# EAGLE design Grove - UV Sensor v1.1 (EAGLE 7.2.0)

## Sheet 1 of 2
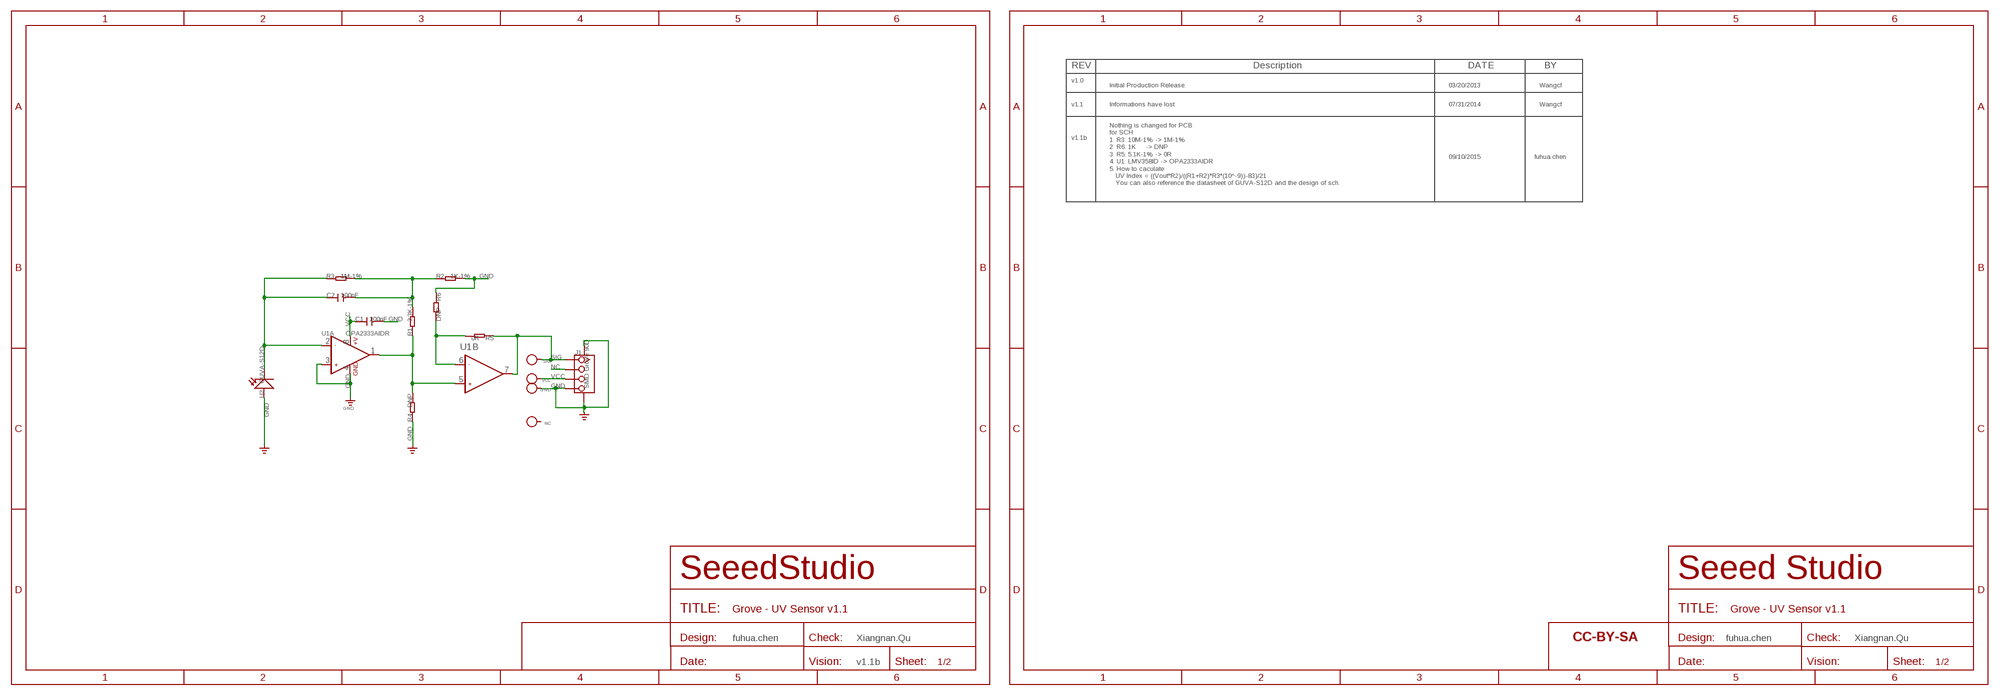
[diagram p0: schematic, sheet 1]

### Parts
C1  100nF  C-0603  [C0603]
C2  100nF  C-0603  [C0603]
GND  PAD-TEST-POINT'4545'  [TP_4545]
J1  SMD Grove 90D  TWIG-4P-2.0-SMD-FEMALE-REINFORCE'DD'  [4P-SMD-2.0]
NC  PAD-TEST-POINT'4545'  [TP_4545]
R1  3.3K-1%  R-0603  [R0603]
R2  1K-1%  R-0603  [R0603]
R3  1M-1%  R-0603  [R0603]
R4  DNP  R-0603  [R0603]
R5  0R  R-0603  [R0603]
R6  DNP  R-0603  [R0603]
SIG  PAD-TEST-POINT'4545'  [TP_4545]
U1  OPA2333AIDR  LMV358D  [SO08]
U2  GUVA-S12D  PHOTODIODE  [LED-3528]
U$30  SEEEDSTUDIO-OPEN-SCH-FRAME  [SEEEDSTUDIO-PCB-FRAME]
VCC  PAD-TEST-POINT'4545'  [TP_4545]

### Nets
GND: C1.2 GND.T J1.4 J1.SS1 J1.SS2 R2.2 R4.1 R6.1 U1.3(A:+IN1) U1.4(A:GND) U2.1(+)
N$1: C2.1 R3.1 U1.2(A:-IN1) U2.2(-)
N$2: R5.2 R6.2 U1.6(B:-IN2)
N$3: C2.2 R1.2 R2.1 R3.2
N$4: J1.1 R5.1 SIG.T U1.7(B:OUT2)
NC: J1.2
SIG: R1.1 R4.2 U1.1(A:OUT1) U1.5(B:+IN2)
VCC: C1.1 J1.3 U1.8(A:+V) VCC.T
Unconnected: NC.T

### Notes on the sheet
- REV | Description | DATE | BY
- v1.0
- Initial Production Release. | 03/20/2013 | Wangcf
- v1.1 | Informations have lost | 07/31/2014 | Wangcf
- v1.1b
- 09/10/2015 | fuhua.chen
- Nothing is changed for PCB
  for SCH:
  1. R3: 10M-1% -> 1M-1%
  2. R6: 1K     -> DNP
  3. R5: 5.1K-1% -> 0R
  4. U1: LMV358ID -> OPA2333AIDR
  5. How to caculate:
     UV Index = ((Vout*R2)/((R1+R2)*R3*(10^-9))-83)/21
     You can also reference the datasheet of GUVA-S12D and the design of sch.
- fuhua.chen | Xiangnan.Qu | fuhua.chen | Xiangnan.Qu
- v1.1b

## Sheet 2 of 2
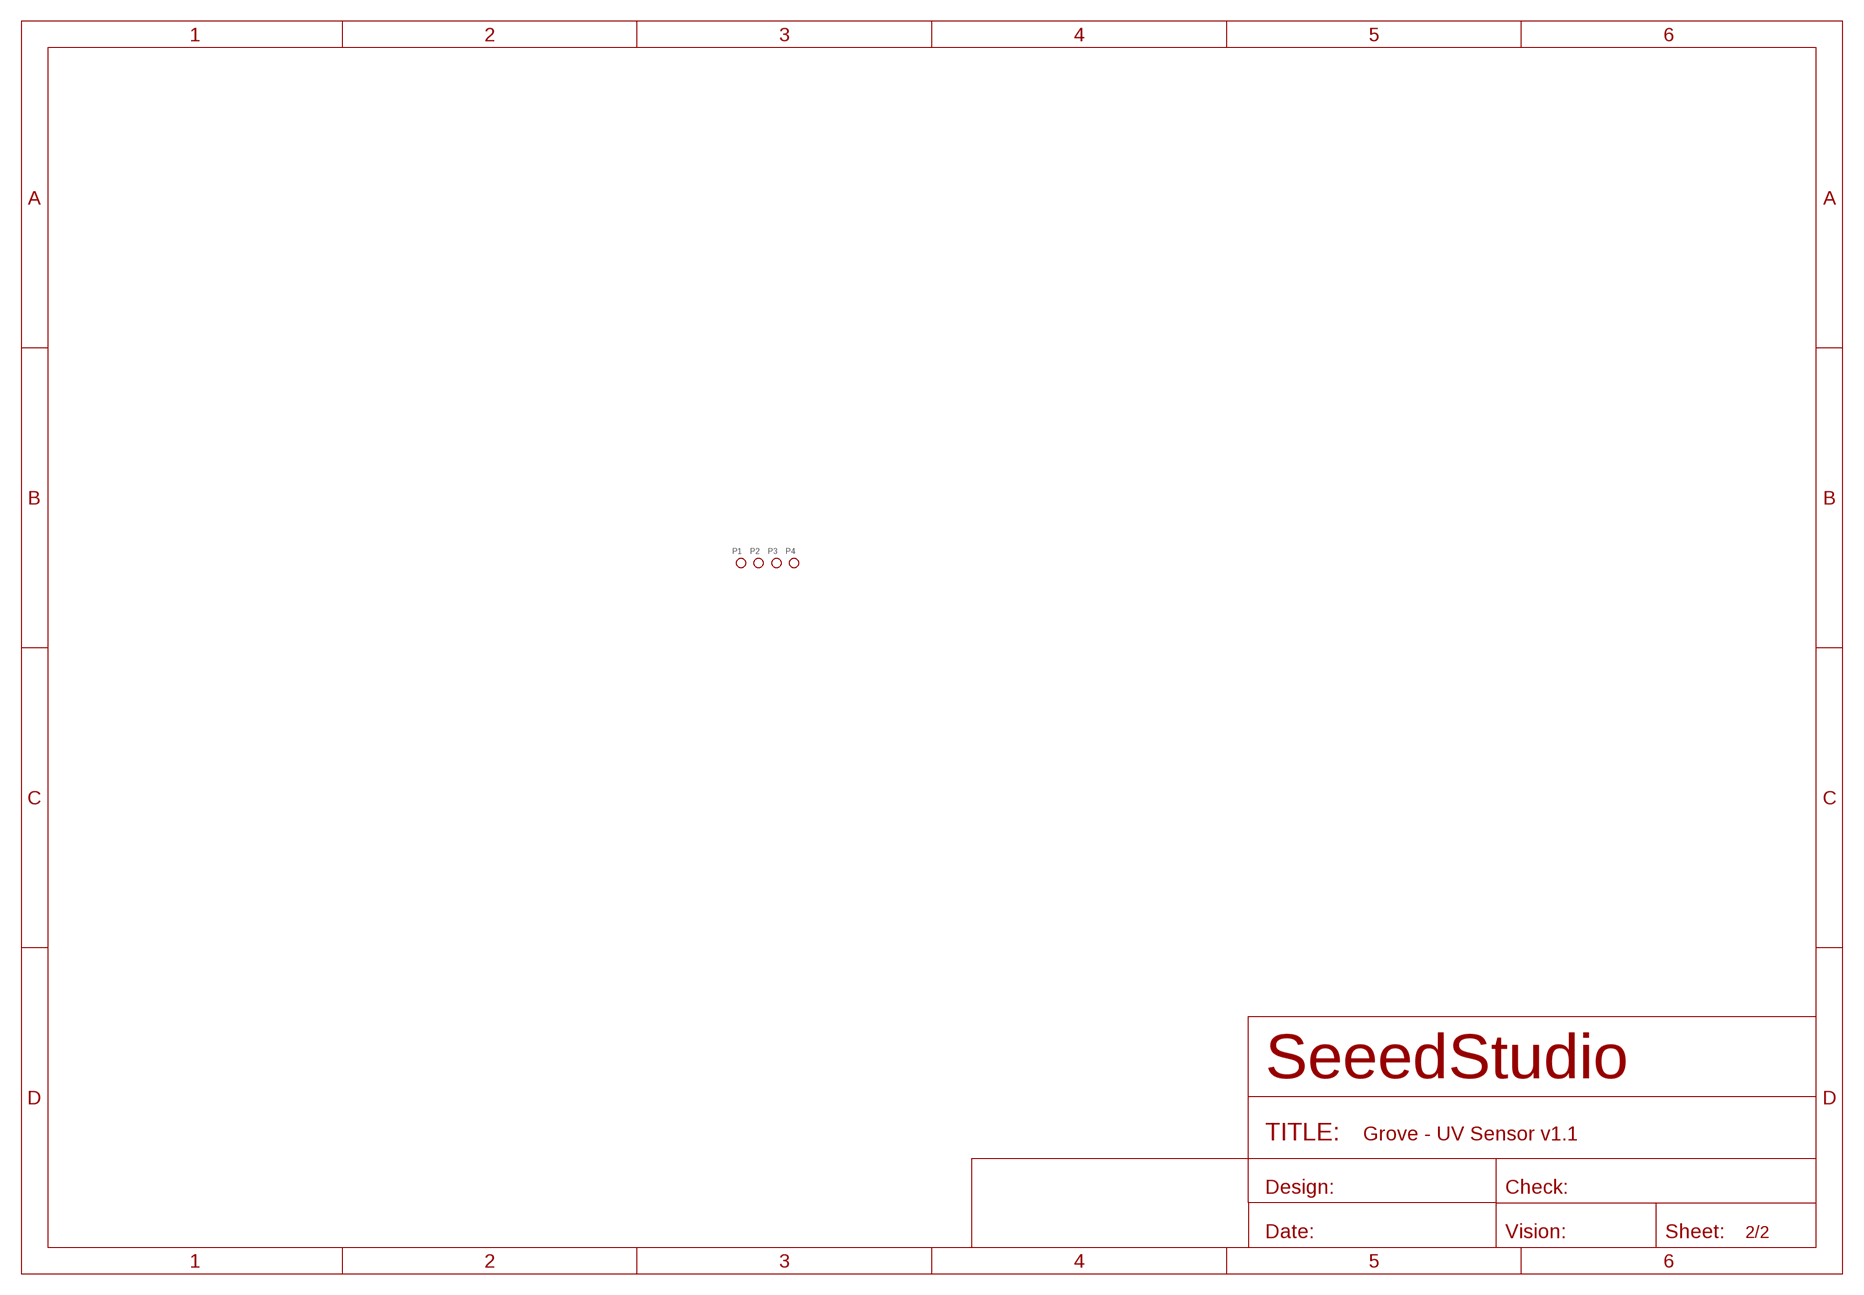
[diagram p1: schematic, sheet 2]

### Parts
P1  PAD-MARK  [ROUND-MARK-1.0]
P2  PAD-MARK  [ROUND-MARK-1.0]
P3  PAD-MARK  [ROUND-MARK-1.0]
P4  PAD-MARK  [ROUND-MARK-1.0]

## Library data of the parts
C1 C2 = Discrete:C*: Ceramic Capacitors
GND NC SIG VCC = Discrete:PAD-TEST-POINT; PARTNO: DNP
J1 = Connector:TWIG-4P-2.0-SMD-FEMALE-REINFORCE
P1-P4 = Discrete:PAD-MARK; PARTNO: DNP
R1-R6 = Discrete:R*
U1 = IC:LMV358: General purpose LOW Voltage, Rail-to-Rail Output Amplifiers http://www.fairchildsemi.com/ds/LM/LMV358.pdf
U2 = Test:PHOTODIODE
U$30 = moudle-new:SEEEDSTUDIO-OPEN-SCH-FRAME

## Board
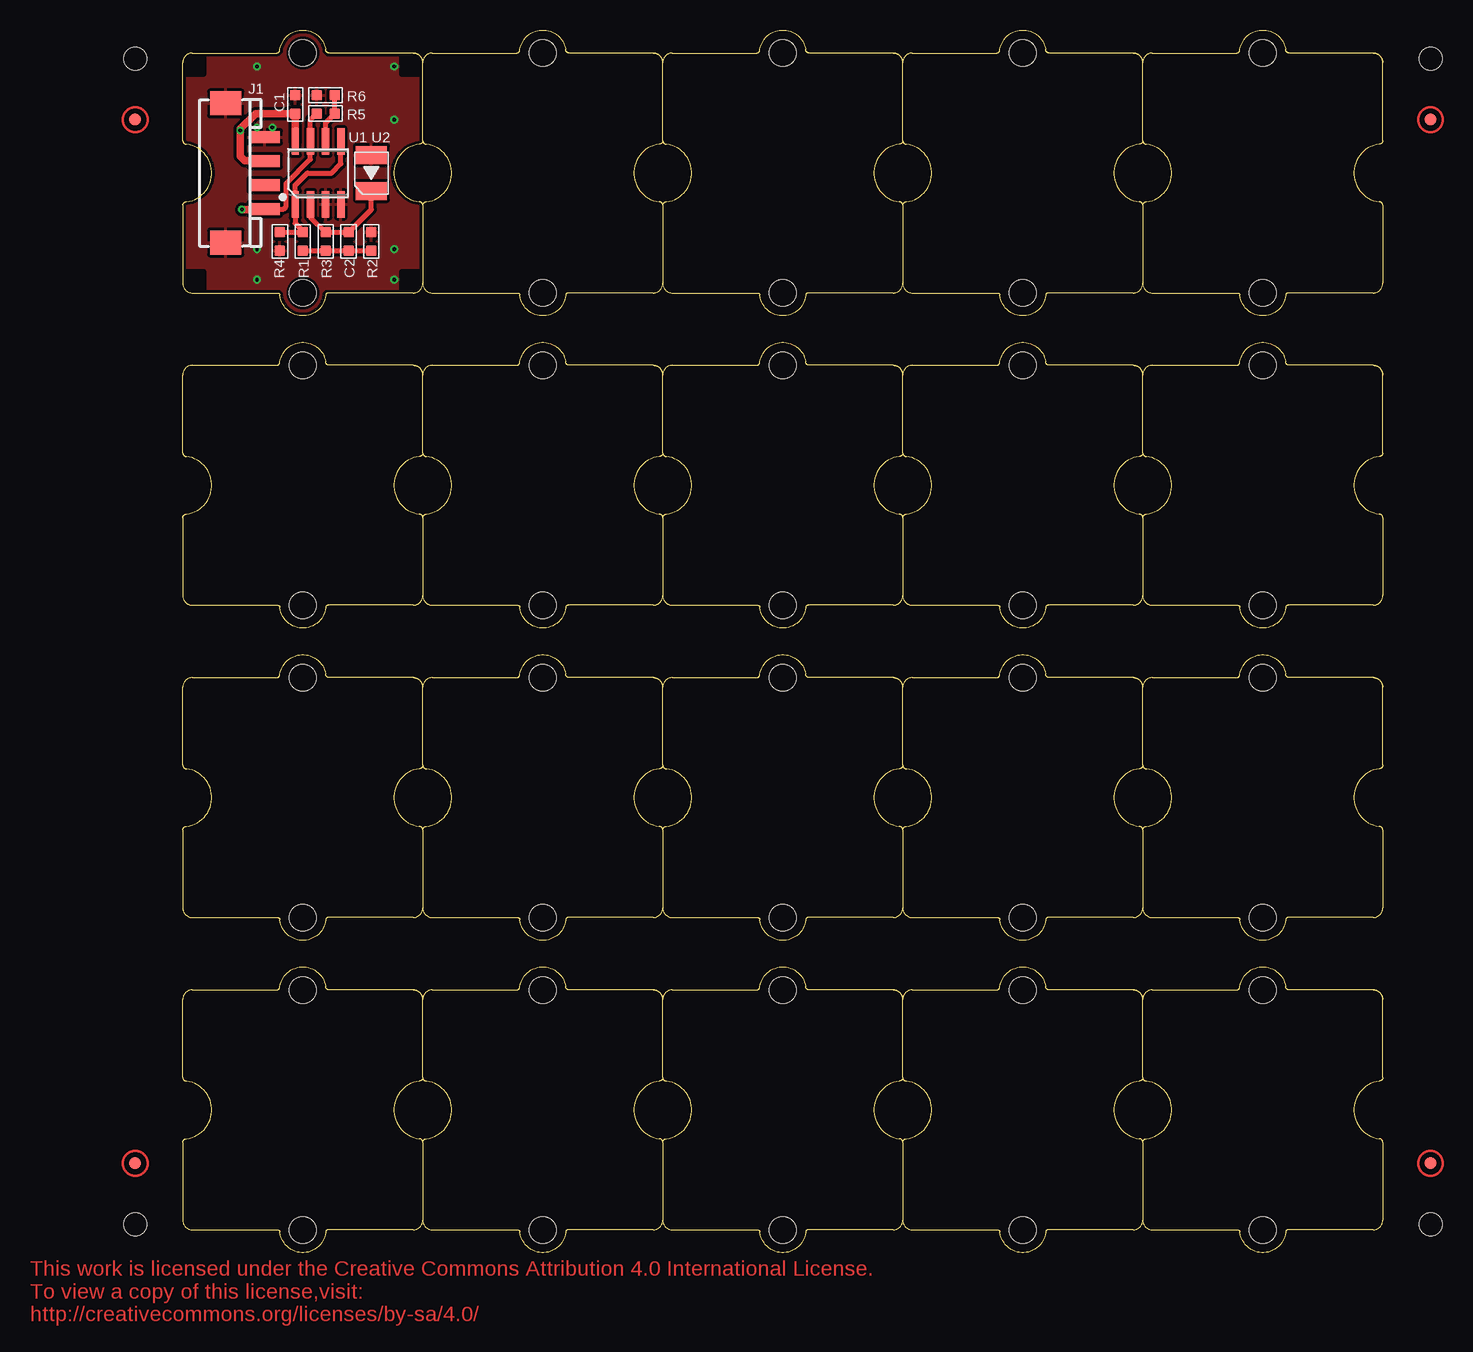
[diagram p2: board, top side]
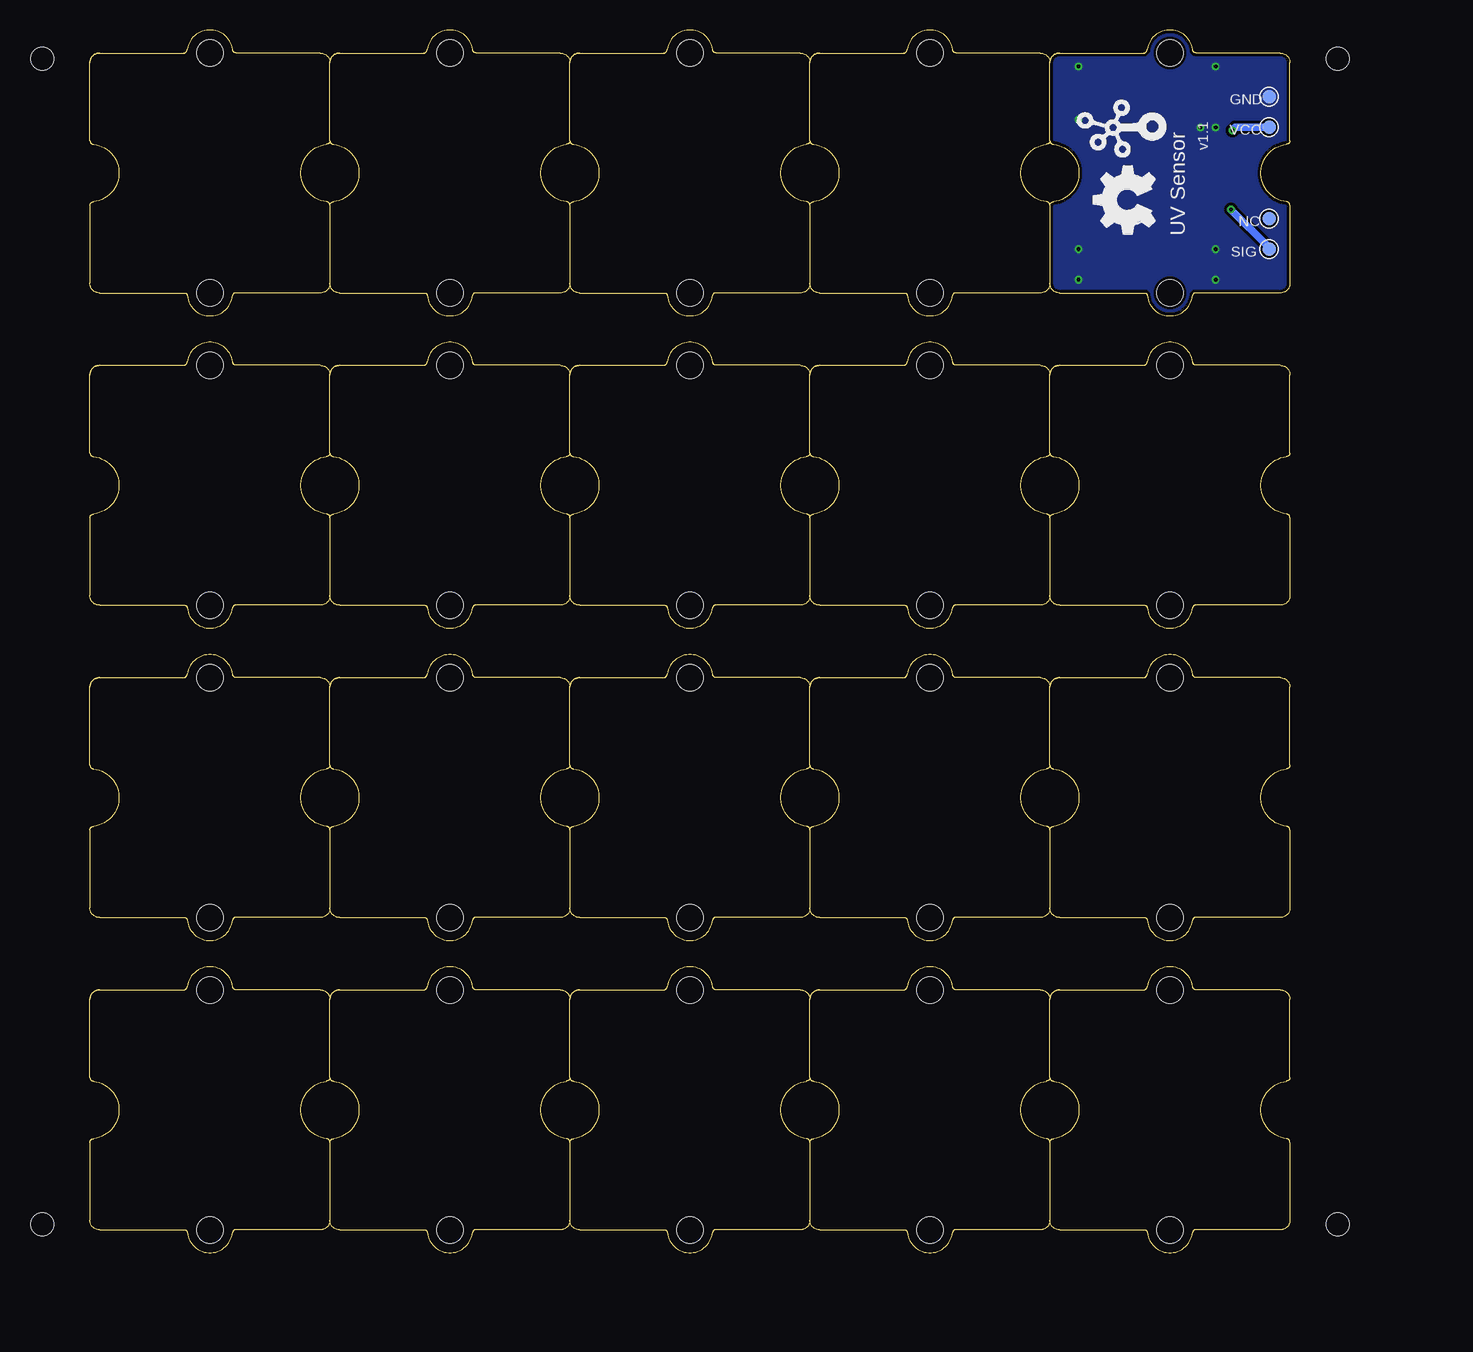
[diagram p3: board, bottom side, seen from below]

Size 100 x 101.93 mm. Coordinates in mm from the lower left corner, seen from the top.
Copper layers (1*16): Top 0.035mm / dielectric 1.5mm / Bottom 0.035mm
Design rules "SeeedStudio_rule_no_angle_090911 *": minimum track width 6mil, minimum drill 12mil, track to track 6mil, track to pad 6mil, pad to pad 6mil, via to via 6mil, smd to smd 0mil, copper to edge 10mil, drill to drill 10mil, minimum pad ring 10mil, minimum via ring 6mil, stop-mask expansion 2mil, vias tented up to drill 25mil, thermal gap 10mil
Holes 1.91 mm at -3.97,2.38 -3.97,99.54 103.98,99.54 103.98,2.38

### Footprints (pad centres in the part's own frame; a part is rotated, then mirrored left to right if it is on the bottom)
C0603 = smd 0.889 x 0.889: 1 -0.762,0; 2 0.762,0
TP_4545 = smd 1.143 x 1.143: T 0,0
4P-SMD-2.0 = smd 1 x 2.54: 1 -3,0; 2 -1,0; 3 1,0; 4 3,0 | smd 2 x 2.6: SS1 -5.8,3.25; SS2 5.8,3.25
ROUND-MARK-1.0 = smd 1.016 x 1.016: P$1 0,0
R0603 = smd 0.889 x 0.889: 1 -0.762,0; 2 0.762,0
SO08 = smd 0.61 x 2.21: 1 -1.905,-2.616; 2 -0.635,-2.616; 3 0.635,-2.616; 4 1.905,-2.616; 5 1.905,2.616; 6 0.635,2.616; 7 -0.635,2.616; 8 -1.905,2.616
LED-3528 = smd 1.5 x 2.6: 1 -1.5,0; 2 1.5,0
1U-DIM-W/-DRILL = hole 2.2: 0,-10; 0,10

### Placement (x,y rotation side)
C1  9.37,95.73 90 top
C2  13.81,84.3 270 top
GND  1.74,96.36 270 bottom
J1  6.83,90.01 90 top
NC  1.74,86.2 270 bottom
P1  not placed on the board
P2  not placed on the board
P3  not placed on the board
P4  not placed on the board
R1  10,84.3 270 top
R2  15.71,84.3 90 top
R3  11.9,84.3 270 top
R4  8.1,84.3 90 top
R5  11.9,94.97 0 top
R6  11.9,96.49 0 top
SIG  1.74,83.66 270 bottom
U1  11.27,90.01 0 top
U2  15.71,90.01 270 top
U$1  [1U-DIM-W/-DRILL]  10,90.01 0 top
U$3  [OSHW_FILLX200_NOTEXT]  11.27,84.93 90 bottom
U$4  [TWIGLOGO]  11.27,93.82 90 bottom
U$10  [1U-DIM-W/-DRILL]  10,90.01 0 top
U$11  [1U-DIM-W/-DRILL]  30,90.01 0 top
U$12  [1U-DIM-W/-DRILL]  50,90.01 0 top
U$13  [1U-DIM-W/-DRILL]  70,90.01 0 top
U$14  [1U-DIM-W/-DRILL]  90,90.01 0 top
U$15  [1U-DIM-W/-DRILL]  30,63.98 0 top
U$16  [1U-DIM-W/-DRILL]  50,63.98 0 top
U$17  [1U-DIM-W/-DRILL]  70,63.98 0 top
U$18  [1U-DIM-W/-DRILL]  90,63.98 0 top
U$19  [1U-DIM-W/-DRILL]  10,63.98 0 top
U$20  [1U-DIM-W/-DRILL]  30,37.94 0 top
U$21  [1U-DIM-W/-DRILL]  50,37.94 0 top
U$22  [1U-DIM-W/-DRILL]  70,37.94 0 top
U$23  [1U-DIM-W/-DRILL]  90,37.94 0 top
U$24  [1U-DIM-W/-DRILL]  10,37.94 0 top
U$25  [1U-DIM-W/-DRILL]  30,11.91 0 top
U$26  [1U-DIM-W/-DRILL]  50,11.91 0 top
U$27  [1U-DIM-W/-DRILL]  70,11.91 0 top
U$28  [1U-DIM-W/-DRILL]  90,11.91 0 top
U$29  [1U-DIM-W/-DRILL]  10,11.91 0 top
U$30  not placed on the board
VCC  1.74,93.82 270 bottom

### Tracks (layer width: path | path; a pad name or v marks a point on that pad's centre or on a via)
GND  (via drill 0.3 pad 0.64)
  other vias: 6.19,93.82 6.19,81.12 6.19,98.9 6.19,83.66 17.62,98.9 17.62,94.46 17.62,81.12 17.62,83.66 7.46,93.82
  pour Top (isolate 0.254): -2.19,102.08 21.43,102.08 21.43,76.68 -2.19,76.68
  pour Bottom (isolate 0.254): -2.19,102.08 -2.19,76.68 21.43,76.68 21.43,102.08
N$1
  Top 0.406: U1.2 10.63,86.33 R3.1 C2.1 15.71,86.97 U2.2
N$2
  Top 0.406: U1.6 11.9,94.2 R5.2 R6.2
N$3
  Top 0.406: R3.2 R1.2 C2.2 R2.1
N$4  (via drill 0.3)
  Top 0.406: R5.1 10.63,94.46 U1.7 10.63,91.16 8.6,89.12 8.6,87.22 8.4,87.01 J1.1
  Top 0.61: v4.92,86.97 6.78,86.97 J1.1
  Bottom 0.61: SIG.T 1.74,83.79 v4.92,86.97
SIG
  Top 0.406: 10,85.19 9.37,85.82 U1.1 9.37,89 10.38,90.01 12.41,90.01 13.18,90.78 U1.5 | 10,85.19 10.13,85.06 | R4.2 9.87,85.06 | 9.87,85.06 10,85.19 | 9.87,85.06 R1.1
VCC  (via drill 0.3)
  Top 0.61: U1.8 C1.1 | 9.37,95.09 C1.1 | C1.1 6.06,94.97 4.79,93.7 v4.79,93.57 4.79,92.68 4.79,91.41 5.17,91.03 6.81,91.03 J1.3
  Bottom 0.61: VCC.T 4.54,93.82 v4.79,93.57

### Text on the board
bPlace: v1.1 | UV Sensor

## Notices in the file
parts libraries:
moudle-new: This work is licensed under the Creative Commons Attribution 4.0 International License.
To view a copy of this license,visit:
http://creativecommons.org/licenses/by-sa/4.0
moudle-new: CC-BY-SA
